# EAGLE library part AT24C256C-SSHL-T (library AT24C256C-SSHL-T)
EEPROM 256K (32K X 8), 2-WI 1.8V Source: Datasheet
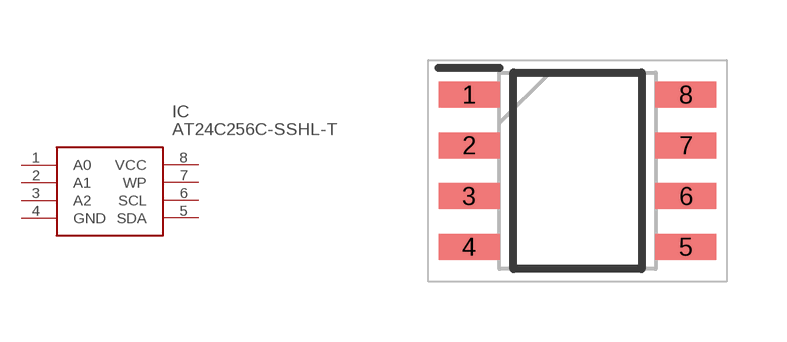
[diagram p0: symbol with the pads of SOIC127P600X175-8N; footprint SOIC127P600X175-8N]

Designator prefix IC

## AT24C256C-SSHL-T (Arrow_Part_Number: AT24C256C-SSHL-T; Arrow_Price-Stock: https://www.arrow.com/en/products/at24c256c-sshl-t/microchip-technology?region=nac; Description: EEPROM 256K (32K X 8), 2-WI 1.8V; Height: 1.75mm; Manufacturer_Name: Microchip; Manufacturer_Part_Number: AT24C256C-SSHL-T; Mouser_Part_Number: 556-AT24C256C-SSHL-T; Mouser_Price-Stock: https://www.mouser.co.uk/ProductDetail/Microchip-Technology-Atmel/AT24C256C-SSHL-T?qs=fzsaQExJLyR3ptk4tHE3tA%3D%3D)  [SOIC127P600X175-8N]
1  A0
2  A1
3  A2
4  GND  pwr
5  SDA
6  SCL
7  WP
8  VCC  pwr

## Footprint SOIC127P600X175-8N (pad centres in mm)
8S1 - JEDEC SOIC
smd 1.525 x 0.65: 1 -2.712,1.905; 2 -2.712,0.635; 3 -2.712,-0.635; 4 -2.712,-1.905; 5 2.712,-1.905; 6 2.712,-0.635; 7 2.712,0.635; 8 2.712,1.905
